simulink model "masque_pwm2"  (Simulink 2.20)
settings: Solver=ode45  StartTime=0.0  StopTime=100  RelTol=1e-3  AbsTol=1e-6
libraries: simulink x1

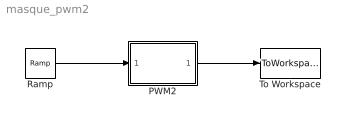
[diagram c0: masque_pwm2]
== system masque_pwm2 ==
  PWM2 : Subsystem  mask(Génération de signal PWM avec entrée le rapport cyclique){T=20, vmax=-.5, vmin=0.5}
      mask prompts: T "période (s)"; vmax "valeur maximale"; vmin "valeur minimale"
      mask help: Ce masque génère un signal PWM dont on peut spécifier la période, les limites hautes et basses. Le rapport cyclique en % est la variable d'entrée du bloc.
  Ramp : simulink/Sources/Ramp  slope=1  start=0  X0=0
  To Workspace : ToWorkspace  VariableName=pwm_var  SampleTime=-1
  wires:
  PWM2/1(PWM) -> To Workspace/1
  Ramp/1 -> PWM2/1(rc)

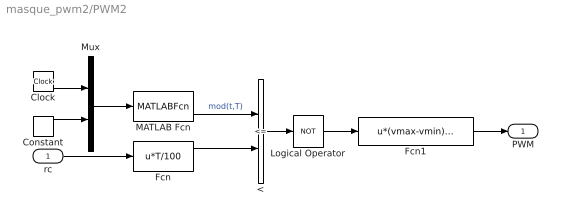
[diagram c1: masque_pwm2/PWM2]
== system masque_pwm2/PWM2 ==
  rc : Inport  Port=1  PortWidth=-1  SampleTime=-1
  < : RelationalOperator  Operator=<=
  Clock : Clock
  Constant : Constant  Value=T
  Fcn : Fcn  Expr=u*T/100
  Fcn1 : Fcn  Expr=u*(vmax-vmin)+vmin
  Logical Operator : Logic  Operator=NOT  Inputs=1
  MATLAB Fcn : MATLABFcn  MATLABFcn=mod(u(1),u(2))  OutputWidth=1
  Mux : Mux  Inputs=2
  PWM : Outport  Port=1  InitialOutput=0
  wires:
  Clock/1 -> Mux/1
  Constant/1 -> Mux/2
  Mux/1 -> MATLAB Fcn/1
  MATLAB Fcn/1 -> </1  "mod(t,T)"
  Fcn/1 -> </2
  Fcn1/1 -> PWM/1
  rc/1 -> Fcn/1
  </1 -> Logical Operator/1
  Logical Operator/1 -> Fcn1/1
